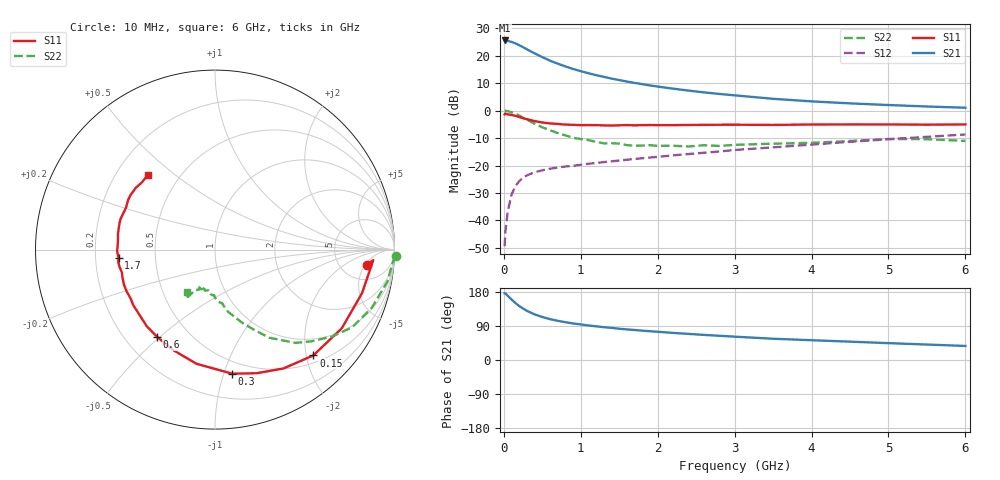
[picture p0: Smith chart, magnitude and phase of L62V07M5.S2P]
!  INFINEON TECHNOLOGIES Small Signal Semiconductors
! BFR380L3 , Si-NPN RF-Transistor in TSLP-3-1
!  Vce=2 V,  Ic=7.5 mA
! Common Emitter S-Parameters:  07. March 2005
#  GHz  S  MA  R  50
! f  S11  S21  S12  S22
! GHz  Mag  Ang  Mag  Ang  Mag  Ang  Mag  Ang
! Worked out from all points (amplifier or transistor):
!   36 points, 10 MHz to 6 GHz, reference 50 ohm
!   highest |S21| = 25.5 dB at 10 MHz (marker M1)
!   |S21| within 3 dB of that: start of sweep to 285 MHz
!   unconditionally stable (mu >= 1): 2.257 GHz to 4.771 GHz
!   at 250 MHz: K = 0.22, MSG = 23.8 dB, |S12| = -24.4 dB
!   at 1.4 GHz: K = 0.84, MSG = 15.1 dB, |S12| = -18.5 dB
!   at 6 GHz: K = 0.96, MSG = 4.9 dB, |S12| = -8.7 dB
!   S11 on the Smith chart (normalised r, x): 10 MHz: 9, -6; 150 MHz: 0.64, -2.14; 300 MHz: 0.40, -1.07; 600 MHz: 0.33, -0.49; 1.7 GHz: 0.30, -0.04; 6 GHz: 0.33, +0.41
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0.01  0.8516 -5.7  18.92 176.1  0.0034 81.2  1.008 -2.1
0.02  0.8837 -3.8  18.84 176.0  0.0062 85.5  0.9917 -4.3
0.05  0.8545 -16.5  18.62 169.5  0.0144 83.1  0.9775 -10.4
0.1  0.8314 -31.8  17.81 159.7  0.0294 74.4  0.9325 -20.2
0.15  0.8049 -47.1  16.79 150.4  0.0421 66.7  0.8786 -29.5
0.2  0.7643 -60.0  15.51 142.3  0.0519 61.9  0.8131 -36.5
0.25  0.727 -71.3  14.27 135.8  0.06 57.1  0.7423 -43.5
0.3  0.6981 -82.1  13.04 129.7  0.0661 53.7  0.6868 -49.2
0.4  0.6444 -99.2  11.03 120.3  0.0756 48.8  0.5763 -58.4
0.5  0.6068 -112.4  9.407 113.5  0.0817 46.2  0.497 -64.0
0.6  0.5839 -123.4  8.114 107.8  0.0875 44.4  0.4382 -69.3
0.7  0.5718 -131.6  7.152 103.5  0.0919 44.3  0.3905 -73.8
0.8  0.5559 -139.3  6.373 99.7  0.0959 43.9  0.3537 -78.2
1.1  0.5447 -154.9  4.785 91.1  0.1076 45.7  0.2906 -86.4
1.4  0.5342 -166.1  3.824 84.7  0.119 47.6  0.2548 -92.2
1.7  0.5392 -174.9  3.19 79.2  0.1316 50.2  0.2291 -99.5
2.2  0.5429 174.6  2.508 71.5  0.153 53.4  0.2291 -104.8
2.8  0.5523 164.1  2.011 63.9  0.1803 56.7  0.2273 -112.5
3.5  0.5482 154.6  1.639 56.1  0.2141 57.6  0.2498 -115.3
4.5  0.5602 146.8  1.354 48.4  0.2703 59.4  0.2792 -118.3
5.5  0.5533 137.5  1.187 40.8  0.333 58.2  0.3014 -121.1
6  0.5599 131.8  1.128 37.1  0.3673 56.8  0.2808 -123.4
